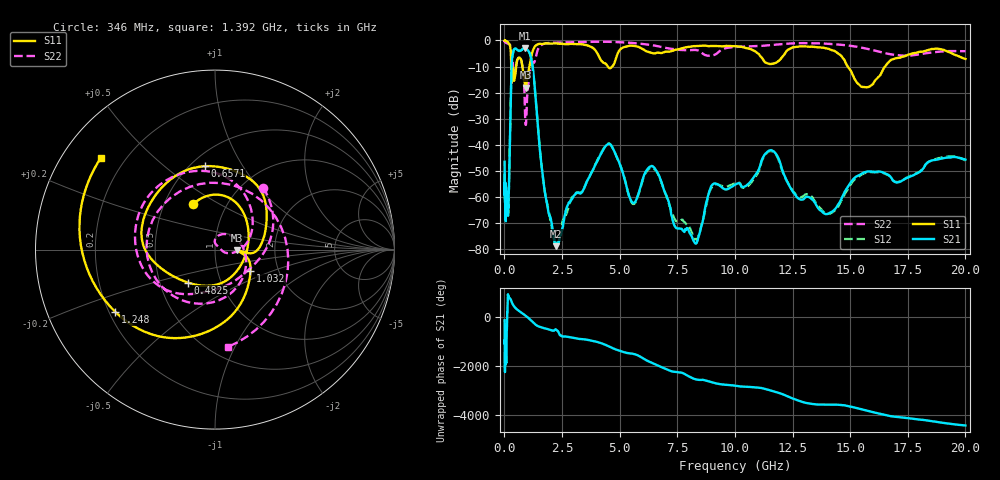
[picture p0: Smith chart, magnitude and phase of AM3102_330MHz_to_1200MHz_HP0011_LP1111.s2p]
! Date/Time: Tue, Sep 11, 2018 5:12 PM
! Network Analyzer: Agilent Technologies E8362B Rev: A.07.50.63
! Sweep from 0.010 to 20.000 GHz, 1601 Points, Sweep Type: LOG
! Power Supply: 4.949 V, 0.001 A
# Hz S DB R 50
!freq MagS11 AngS11 MagS21 AngS21 MagS12 AngS12 MagS22 AngS22
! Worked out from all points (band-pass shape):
!   1601 points, 10 MHz to 20 GHz, reference 50 ohm
!   highest |S21| = -2.98 dB at 886.4 MHz (marker M1); lowest = -79.0 dB at 2.238 GHz (marker M2)
!   |S21| within 3 dB of the highest: 347.9 MHz to 1.138 GHz (790.2 MHz wide, 106 % of centre)
!   lowest |S11| = -18.1 dB at 920.7 MHz (marker M3), VSWR 1.28, Z = 64.2 - j0.618 ohm
!   |S11| at or under -10 dB: 298.8 MHz to 510.3 MHz (211.6 MHz wide, 52.3 % of centre); 780.6 MHz to 1.086 GHz (305.8 MHz wide, 32.8 % of centre); 14.89 GHz to 16.51 GHz (1.621 GHz wide, 10.3 % of centre)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
!   |S22| runs from -32.4 to -0.3 dB; largest |S21 - S12| = 0.013
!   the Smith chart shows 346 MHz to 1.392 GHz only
!   S11 on the Smith chart (normalised r, x): 346 MHz: 0.70, +0.38; 482.5 MHz: 0.70, -0.27; 657.1 MHz: 0.59, +0.70; 1.032 GHz: 1.44, -0.37; 1.248 GHz: 0.23, -0.27; 1.392 GHz: 0.11, +0.35
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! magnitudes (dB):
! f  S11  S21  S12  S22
! 10 MHz  0.0  -46.6  -51.5  -0.3
! 35.55 MHz  0.0  -62.8  -62.4  -0.6
! 126.4 MHz  -0.4  -63.9  -64.1  -1.1
! 179.6 MHz  -0.9  -62.7  -61.5  -1.3
! 346 MHz  -11.0  -6.1  -6.2  -7.2
! 447.2 MHz  -14.4  -3.2  -3.2  -13.5
! 482.5 MHz  -12.5  -3.1  -3.1  -12.0
! 657.1 MHz  -6.6  -3.9  -4.1  -6.5
! 886.4 MHz  -16.8  -3.0  -3.0  -24.9
! 920.7 MHz  -18.1  -3.0  -3.1  -32.3
! 1.032 GHz  -12.7  -3.9  -3.9  -17.3
! 1.248 GHz  -3.7  -11.6  -11.7  -8.5
! 1.392 GHz  -1.8  -26.0  -26.4  -5.2
! 1.59 GHz  -1.3  -46.2  -46.2  -1.8
! 2.238 GHz  -1.1  -79.0  -77.8  -0.8
! 4.457 GHz  -9.7  -40.0  -39.9  -0.5
! 5.652 GHz  -2.1  -62.2  -62.6  -1.0
! 6.457 GHz  -4.9  -48.5  -49.0  -1.9
! 8.188 GHz  -2.2  -76.5  -75.3  -3.7
! 11.47 GHz  -8.9  -42.4  -42.6  -1.9
! 14.01 GHz  -3.1  -66.6  -66.6  -1.3
! 20 GHz  -7.1  -45.7  -46.0  -4.1
